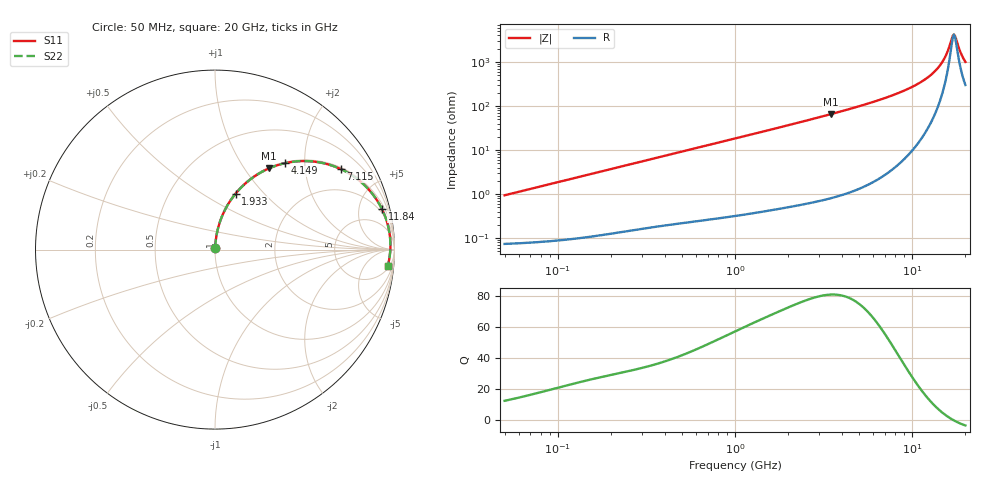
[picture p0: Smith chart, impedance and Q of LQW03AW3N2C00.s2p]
!Murata Part Number: LQW03AW3N2C00
!These Parameters are Measured in Series Mode Connection
!  o--[Z]--o
!Port1  Port2
!  o-------o
!Freq. Start=50[MHz] Stop=20[GHz], 401[Steps]
# Hz S RI R 50
!Freq.(Hz) S11(Real) S11(Imag) S21(Real) S21(Imag) S12(Real) S12(Imag) S22(Real) S22(Imag)
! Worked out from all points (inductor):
!   401 points, 50 MHz to 20 GHz, reference 50 ohm
!   read as one part in series: L = 2.99 nH near 51.52 MHz
!   highest Q = 81 at 3.467 GHz (marker M1), where L = 2.99 nH
!   self-resonance near 17.22 GHz
!   S11 on the Smith chart (normalised r, x): 50 MHz: 1.00, +0.02; 1.933 GHz: 1.01, +0.71; 4.149 GHz: 1.02, +1.59; 7.115 GHz: 1.06, +3.09; 11.84 GHz: 1.49, +8.05; 20 GHz: 7, -19
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5e7  0.000828 0.00938  0.9992 -0.00938  0.9992 -0.00938  0.000828 0.00938
1.364002e8  0.00166 0.0254  0.9983 -0.0254  0.9983 -0.0254  0.00166 0.0254
3.721004e8  0.0065 0.0679  0.9935 -0.0679  0.9935 -0.0679  0.0065 0.0679
1e9  0.0351 0.1756  0.9649 -0.1756  0.9649 -0.1756  0.0351 0.1756
1.932977e9  0.115 0.3122  0.885 -0.3122  0.885 -0.3122  0.115 0.3122
2.728004e9  0.2067 0.3986  0.7933 -0.3986  0.7933 -0.3986  0.2067 0.3986
3.466789e9  0.3008 0.4525  0.6992 -0.4525  0.6992 -0.4525  0.3008 0.4525
4.149438e9  0.3885 0.4812  0.6115 -0.4812  0.6115 -0.4812  0.3885 0.4812
5.515528e9  0.5505 0.4905  0.4495 -0.4905  0.4495 -0.4905  0.5505 0.4905
7.114996e9  0.7017 0.4485  0.2983 -0.4485  0.2983 -0.4485  0.7017 0.4485
7.442007e9  0.7272 0.4358  0.2728 -0.4358  0.2728 -0.4358  0.7272 0.4358
9.600142e9  0.855 0.3364  0.145 -0.3364  0.145 -0.3364  0.855 0.3364
1.183995e10  0.9299 0.2267  0.0701 -0.2267  0.0701 -0.2267  0.9299 0.2267
1.334722e10  0.9576 0.1568  0.0424 -0.1568  0.0424 -0.1568  0.9576 0.1568
1.460232e10  0.9706 0.1024  0.0294 -0.1024  0.0294 -0.1024  0.9706 0.1024
1.550395e10  0.9755 0.0656  0.0245 -0.0656  0.0245 -0.0656  0.9755 0.0656
1.670968e10  0.9774 0.0196  0.0226 -0.0196  0.0226 -0.0196  0.9774 0.0196
1.721783e10  0.9769 0.00123  0.0231 -0.00123  0.0231 -0.00123  0.9769 0.00123
1.747767e10  0.9763 -0.00792  0.0237 0.00792  0.0237 0.00792  0.9763 -0.00792
1.774144e10  0.9756 -0.017  0.0244 0.017  0.0244 0.017  0.9756 -0.017
1.912117e10  0.9691 -0.0622  0.0309 0.0622  0.0309 0.0622  0.9691 -0.0622
2e10  0.963 -0.0888  0.037 0.0888  0.037 0.0888  0.963 -0.0888
